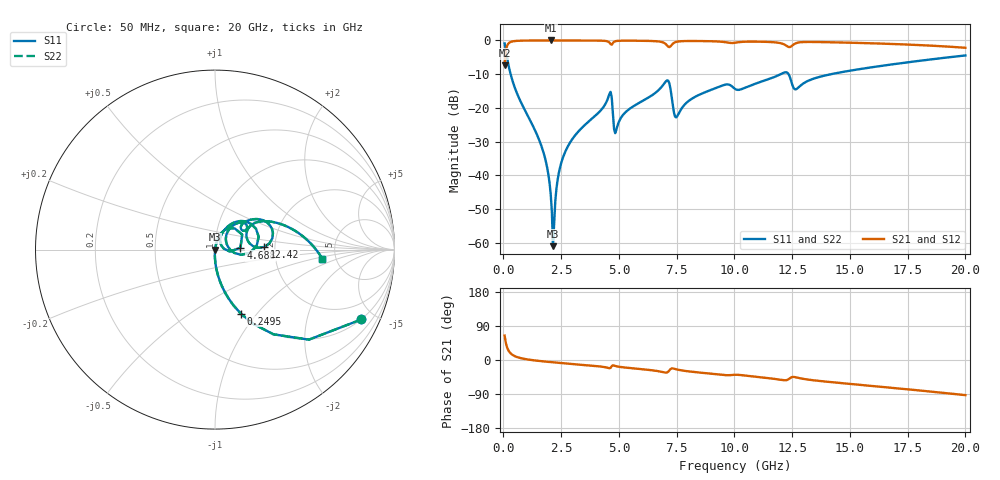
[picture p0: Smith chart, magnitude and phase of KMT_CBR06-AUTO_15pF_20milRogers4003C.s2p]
! Data measured by Modelithics Inc. support@modelithics.com 813-866-6335
! KEMET CBR06-AUTO 15pF, Pad Width= 0.851mm, Pad Length= 0.64mm, Pad Gap= 0.62mm, 20mil Rogers 4003C substrate Data, January 2022
# hz S ma R 50
! 2 Port Network Data from SP1.SP block
! freq  magS11  angS11  magS21  angS21  magS12  angS12  magS22  angS22
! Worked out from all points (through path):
!   401 points, 50 MHz to 20 GHz, reference 50 ohm
!   highest |S21| = -0.01 dB at 2.045 GHz (marker M1); lowest = -7.4 dB at 50 MHz (marker M2)
!   group delay of S21, straight-line fit = 13.4 ps
!   lowest |S11| = -61.0 dB at 2.145 GHz (marker M3), VSWR 1.00, Z = 50.1 - j0.0574 ohm
!   |S11| at or under -10 dB: 310.1 MHz to 12 GHz (11.69 GHz wide, 190 % of centre); 12.34 GHz to 14.18 GHz (1.84 GHz wide, 13.9 % of centre)
!   |S22| runs from -61.0 to -0.9 dB; largest |S21 - S12| = 0
!   S11 on the Smith chart (normalised r, x): 50 MHz: 0.99, -4.19; 249.5 MHz: 0.99, -0.83; 4.688 GHz: 1.33, +0.03; 12.42 GHz: 1.76, +0.06; 20 GHz: 3.89, -0.61
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5e7  0.9032 -25.5  0.4288 64.4  0.4288 64.4  0.9032 -25.5
2.495e8  0.3846 -68.0  0.9227 21.9  0.9227 21.9  0.3846 -68.0
6.98375e8  0.1341 -84.1  0.9905 5.7  0.9905 5.7  0.1341 -84.1
1.695875e9  0.02409 -91.9  0.999 -3.5  0.999 -3.5  0.02409 -91.9
1.94525e9  0.01031 -91.1  0.9992 -5.0  0.9992 -5.0  0.01031 -91.1
2.045e9  0.005329 -87.8  0.9992 -5.5  0.9992 -5.5  0.005329 -87.8
2.14475e9  0.0008941 -39.9  0.9992 -6.1  0.9992 -6.1  0.0008941 -39.9
2.54375e9  0.01703 79.0  0.9989 -8.2  0.9989 -8.2  0.01703 79.0
3.391625e9  0.05056 76.1  0.9975 -12.6  0.9975 -12.6  0.05056 76.1
4.588625e9  0.1614 46.8  0.9295 -21.7  0.9295 -21.7  0.1614 46.8
4.688375e9  0.1424 4.2  0.8651 -16.2  0.8651 -16.2  0.1424 4.2
4.887875e9  0.04741 50.5  0.9803 -16.4  0.9803 -16.4  0.04741 50.5
6.73325e9  0.186 54.6  0.9643 -29.8  0.9643 -29.8  0.186 54.6
7.13225e9  0.2536 16.2  0.8101 -31.0  0.8101 -31.0  0.2536 16.2
7.481375e9  0.07242 25.7  0.9518 -24.5  0.9518 -24.5  0.07242 25.7
8.52875e9  0.1596 53.8  0.9791 -33.4  0.9791 -33.4  0.1596 53.8
1.0025e10  0.1913 33.2  0.924 -38.9  0.924 -38.9  0.1913 33.2
1.2419e10  0.2758 3.1  0.8012 -47.3  0.8012 -47.3  0.2758 3.1
1.266838e10  0.1891 21.5  0.9112 -45.8  0.9112 -45.8  0.1891 21.5
1.336662e10  0.2668 33.8  0.949 -53.1  0.949 -53.1  0.2668 33.8
1.670825e10  0.436 16.0  0.8897 -72.7  0.8897 -72.7  0.436 16.0
2e10  0.5996 -4.8  0.7781 -92.7  0.7781 -92.7  0.5996 -4.8
